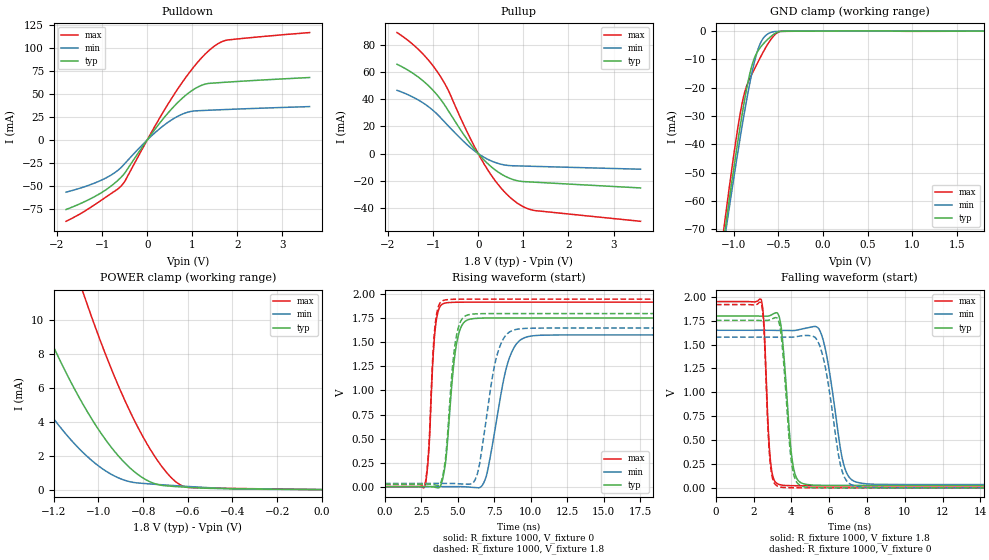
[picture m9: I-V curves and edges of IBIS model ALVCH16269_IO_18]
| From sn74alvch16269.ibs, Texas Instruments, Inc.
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[Model]   ALVCH16269_IO_18
Model_type  3-state
Enable   Active-Low
Vref =   0
Rref =   1000
Cref =   30p
Vmeas =   0.9
| variable   typ   min   max
C_comp   7.92pF   7.07pF   8.91pF
| C_pullup   9.02pF   7.62pF   9.78pF
| C_pulldown   9.61pF   7.92pF   12.09pF
| C_tri-state   7.92pF   7.07pF   8.91pF
[Temperature Range]   40   100   -40
| Ambient temperature   25   85   -40
[Voltage range]   1.8   1.65   1.95
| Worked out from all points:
|   slope of the pulldown table from 0 to 0.27 V, typ, clamps not added: 15.1 ohm
|   slope of the pullup table from 0 to 0.27 V, typ, clamps not added: 29.6 ohm
|   GND clamp passes 1 mA (typ) near -0.54 V on its own axis
|   POWER clamp passes 1 mA (typ) near -0.83 V on its own axis
|   rising waveform, R_fixture 1000, V_fixture 0: 20-80 % time 599ps typ, 1.15ns min, 373ps max; typ from 0 V to 1.75 V
|   falling waveform, R_fixture 1000, V_fixture 1.8: 20-80 % time 411ps typ, 724ps min, 255ps max; typ from 1.8 V to 0.026 V
|   rising waveform, R_fixture 1000, V_fixture 1.8: 20-80 % time 565ps typ, 1ns min, 364ps max; typ from 0.026 V to 1.8 V
|   falling waveform, R_fixture 1000, V_fixture 0: 20-80 % time 403ps typ, 724ps min, 252ps max; typ from 1.75 V to 0 V
[GND Clamp]
| ALVCH16269_IO_18
|   Voltage   I(typ)   I(min)   I(max)
-1.8V     -241mA     -232.5mA   -248.3mA
-1.125V   -76.67mA   -78.48mA   -73.38mA
-1.095V   -69.81mA   -72.03mA   -66.09mA
-1.08V    -66.41mA   -68.83mA   -62.49mA
-925mV    -33.16mA   -37.21mA   -28.73mA
-880mV    -24.66mA   -28.78mA   -21.99mA
-825mV    -15.81mA   -19.28mA   -17.07mA
-780mV    -10.59mA   -12.52mA   -14.16mA
-720mV    -6.609mA   -5.769mA   -10.44mA
-610mV    -2.66mA    -859uA     -4.199mA
-470mV    -90.33uA   -98.91uA   -118.2uA
1.8V      44.19pA    9.86uA     -22.55uA
[POWER Clamp]
| ALVCH16269_IO_18
|   Voltage   I(typ)   I(min)   I(max)
-1.8V     30.34mA    19.02mA    49.01mA
-1.53V    19.35mA    11.38mA    33.41mA
-1.3V     11.34mA    6.043mA    21.61mA
-1.17V    7.533mA    3.651mA    15.72mA
-1.06V    4.805mA    2.064mA    11.25mA
-990mV    3.342mA    1.297mA    8.694mA
-915mV    2.044mA    715.7uA    6.233mA
-835mV    1.006mA    405.9uA    3.96mA
-755mV    381.1uA    320.1uA    2.096mA
-685mV    209.8uA    256.9uA    856.6uA
-630mV    157.6uA    210.3uA    252.4uA
-16.28fV  44.19pA    278.2pA    7.565pA
[Pulldown]
| ALVCH16269_IO_18
|   Voltage   I(typ)   I(min)   I(max)
-1.8V     -75.27mA   -56.5mA    -88.02mA
-1.05V    -58.08mA   -44.24mA   -66.32mA
-760mV    -48.26mA   -36.71mA   -56.63mA
-550mV    -38.84mA   -28.37mA   -48.29mA
130mV     8.835mA    6.032mA    11.4mA
635mV     38.47mA    24.53mA    52.14mA
865mV     48.86mA    29.58mA    68.42mA
1.075V    56.07mA    31.57mA    81.67mA
1.265V    60.22mA    32.01mA    92mA
1.455V    61.62mA    32.42mA    100.4mA
1.78V     62.69mA    33.08mA    108.3mA
3.6V      67.66mA    36.18mA    116.3mA
[Pullup]
| ALVCH16269_IO_18
|   Voltage   I(typ)   I(min)   I(max)
-1.8V     65.73mA    46.56mA    89.05mA
-1.315V   55.97mA    39.2mA     76.3mA
-1.105V   50.03mA    34.56mA    68.86mA
-915mV    43.31mA    29.2mA     60.66mA
-680mV    32.44mA    20.97mA    47.7mA
-240mV    10.19mA    6.363mA    15.59mA
125mV     -4.565mA   -2.634mA   -7.325mA
460mV     -13.97mA   -7.421mA   -23.49mA
800mV     -19.37mA   -8.976mA   -34.81mA
1.03V     -20.65mA   -9.192mA   -39.55mA
1.26V     -21.06mA   -9.405mA   -41.95mA
3.6V      -25.27mA   -11.49mA   -49.82mA
[Ramp]
| ALVCH16269_IO_18
| variable   typ   min   max
dV/dt_r   1.06/6.08E-10   0.95/1.15E-09   1.16/3.85E-10
dV/dt_f   1.08/4.24E-10   0.99/7.47E-10   1.17/2.60E-10
R_load = 1000
[Rising Waveform]
| ALVCH16269_IO_18
R_fixture =   1000
C_fixture =   0
L_fixture =   0
V_fixture =   0
V_fixture_min = 0
V_fixture_max = 0
|   Time   V(typ)   V(min)   V(max)
0s        71.64pV    3.177nV    54.75pV
2.75ns    1.894mV    -188.4uV   5.55mV
3.46ns    -6.893mV   882.9uV    1.651V
4.11ns    199.9mV    280.1uV    1.908V
4.895ns   1.471V     333.8uV    1.917V
5.84ns    1.742V     -5.285mV   1.919V
6.86ns    1.753V     69.33mV    1.919V
8.415ns   1.754V     1.285V     1.919V
9.805ns   1.754V     1.56V      1.919V
50ns      1.754V     1.578V     1.919V
[Falling Waveform]
| ALVCH16269_IO_18
R_fixture =   1000
C_fixture =   0
L_fixture =   0
V_fixture =   1.8
V_fixture_min = 1.65
V_fixture_max = 1.95
|   Time   V(typ)   V(min)   V(max)
0s        1.8V       1.65V      1.95V
2.405ns   1.798V     1.65V      1.971V
2.9ns     1.807V     1.65V      265.9mV
3.47ns    1.663V     1.648V     29.87mV
4.075ns   248.2mV    1.647V     22.79mV
4.79ns    35.5mV     1.673V     21.86mV
5.6ns     26.7mV     1.6V       21.72mV
6.76ns    25.71mV    250.5mV    21.69mV
7.64ns    25.6mV     50.79mV    21.69mV
50ns      25.55mV    33.84mV    21.68mV
[Rising Waveform]
| ALVCH16269_IO_18
R_fixture =   1000
C_fixture =   0
L_fixture =   0
V_fixture =   1.8
V_fixture_min = 1.65
V_fixture_max = 1.95
|   Time   V(typ)   V(min)   V(max)
0s        25.55mV    33.84mV    21.68mV
2.75ns    27.38mV    33.63mV    27.79mV
3.445ns   18.67mV    34.9mV     1.683V
4.065ns   195.3mV    33.7mV     1.939V
4.84ns    1.512V     32.63mV    1.949V
5.74ns    1.788V     25.35mV    1.95V
6.415ns   1.798V     180.4mV    1.95V
7.735ns   1.8V       1.394V     1.95V
8.945ns   1.8V       1.633V     1.95V
50ns      1.8V       1.65V      1.95V
[Falling Waveform]
| ALVCH16269_IO_18
R_fixture =   1000
C_fixture =   0
L_fixture =   0
V_fixture =   0
V_fixture_min = 0
V_fixture_max = 0
|   Time   V(typ)   V(min)   V(max)
0s        1.754V     1.578V     1.919V
2.405ns   1.752V     1.578V     1.935V
2.885ns   1.761V     1.578V     248.4mV
3.43ns    1.639V     1.577V     8.079mV
4.03ns    232.5mV    1.578V     1.001mV
4.72ns    9.26mV     1.596V     156.9uV
5.53ns    821.9uV    1.47V      24.66uV
6.64ns    103.7uV    205.5mV    4.706uV
7.515ns   31.72uV    12.98mV    2.573uV
50ns      555nV      984.4nV    310.9nV
